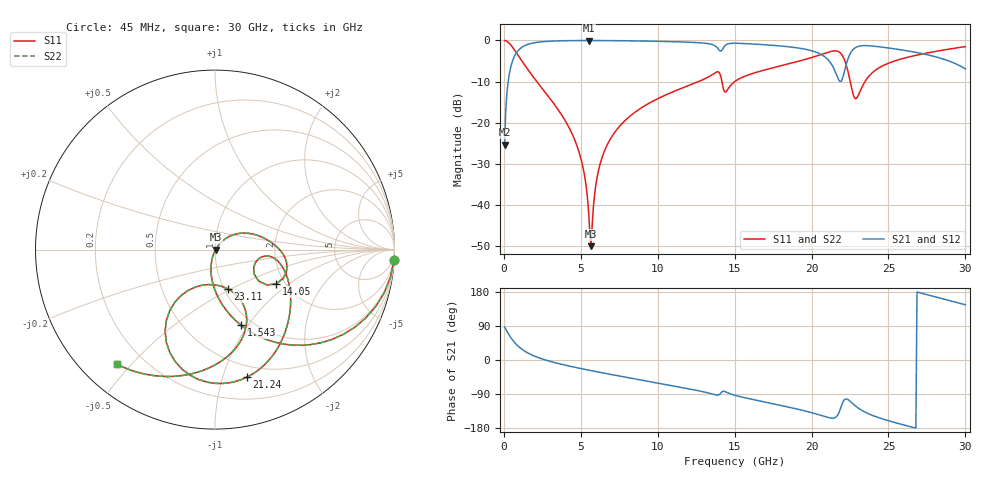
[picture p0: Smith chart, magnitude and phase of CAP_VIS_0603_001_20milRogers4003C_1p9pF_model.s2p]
! S-parameter model data by Modelithics Inc.  support@modelithics.com  813-866-6335  Tampa FL USA
! S-Parameter data specifications:
! Substrate: 20-mil Rogers 4003C, substrate thickness, H=0.508mm, Dielectric constant, Er=3.75
! PCB Mounting Pad Footprint: Pad width, PadW=0.90mm , Pad length, PadL=1.00mm , Pad gap, PadG (edge-to-edge)=1.00mm , Reference planes=3.0mm apart
! Created Wed Nov 18 13:19:21 2015
# hz S ma R 50
! 2 Port Network Data from SP1.SP block
! freq  magS11  angS11  magS21  angS21  magS12  angS12  magS22  angS22
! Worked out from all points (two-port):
!   401 points, 45 MHz to 30 GHz, reference 50 ohm
!   highest |S21| = -0.03 dB at 5.512 GHz (marker M1); lowest = -25.3 dB at 45 MHz (marker M2)
!   |S21| within 3 dB of the highest: 811.4 MHz to 20.41 GHz (19.6 GHz wide, 185 % of centre); 22.54 GHz to 26.96 GHz (4.42 GHz wide, 17.9 % of centre)
!   lowest |S11| = -50.0 dB at 5.662 GHz (marker M3), VSWR 1.01, Z = 50.3 - j0.0801 ohm
!   |S11| at or under -10 dB: 2.14 GHz to 12.65 GHz (10.51 GHz wide, 142 % of centre); 14.17 GHz to 15.01 GHz (833.3 MHz wide, 5.71 % of centre); 22.51 GHz to 23.47 GHz (959.5 MHz wide, 4.17 % of centre)
!   |S22| runs from -50.0 to 0.0 dB; largest |S21 - S12| = 0
!   S11 on the Smith chart (normalised r, x): 45 MHz: 1, -34; 1.543 GHz: 0.88, -0.93; 14.05 GHz: 1.80, -0.81; 21.24 GHz: 0.39, -1.20; 23.11 GHz: 1.04, -0.48; 30 GHz: 0.10, -0.46
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4.5e7  0.9985 -3.3  0.05419 86.7  0.05419 86.7  0.9985 -3.3
4.94325e8  0.8571 -33.4  0.5147 56.5  0.5147 56.5  0.8571 -33.4
1.54275e9  0.446 -71.0  0.8935 18.9  0.8935 18.9  0.446 -71.0
4.014038e9  0.1037 -102.5  0.9917 -13.9  0.9917 -13.9  0.1037 -102.5
5.062462e9  0.0333 -108.1  0.9961 -23.1  0.9961 -23.1  0.0333 -108.1
5.511788e9  0.008023 -94.5  0.9965 -26.8  0.9965 -26.8  0.008023 -94.5
5.661562e9  0.003177 -14.5  0.9964 -28.0  0.9964 -28.0  0.003177 -14.5
6.110888e9  0.02443 50.8  0.9959 -31.6  0.9959 -31.6  0.02443 50.8
6.784875e9  0.05723 49.8  0.9943 -36.8  0.9943 -36.8  0.05723 49.8
1.007992e10  0.1994 27.3  0.9744 -61.4  0.9744 -61.4  0.1994 27.3
1.300054e10  0.3381 3.6  0.9272 -84.2  0.9272 -84.2  0.3381 3.6
1.404896e10  0.3909 -29.2  0.7466 -89.7  0.7466 -89.7  0.3909 -29.2
1.44234e10  0.2367 -17.5  0.8811 -84.2  0.8811 -84.2  0.2367 -17.5
1.50225e10  0.3181 -7.4  0.924 -93.2  0.924 -93.2  0.3181 -7.4
2.003996e10  0.622 -52.7  0.7457 -139.4  0.7457 -139.4  0.622 -52.7
2.123816e10  0.7328 -76.0  0.5335 -153.2  0.5335 -153.2  0.7328 -76.0
2.183726e10  0.7146 -101.0  0.3172 -133.0  0.3172 -133.0  0.7146 -101.0
2.22117e10  0.5322 -121.5  0.4785 -103.1  0.4785 -103.1  0.5322 -121.5
2.273591e10  0.2115 -110.1  0.7874 -117.1  0.7874 -117.1  0.2115 -110.1
2.311035e10  0.2314 -71.7  0.8532 -129.0  0.8532 -129.0  0.2314 -71.7
2.505742e10  0.5338 -74.9  0.8065 -160.9  0.8065 -160.9  0.5338 -74.9
3e10  0.8404 -130.6  0.4512 145.7  0.4512 145.7  0.8404 -130.6
